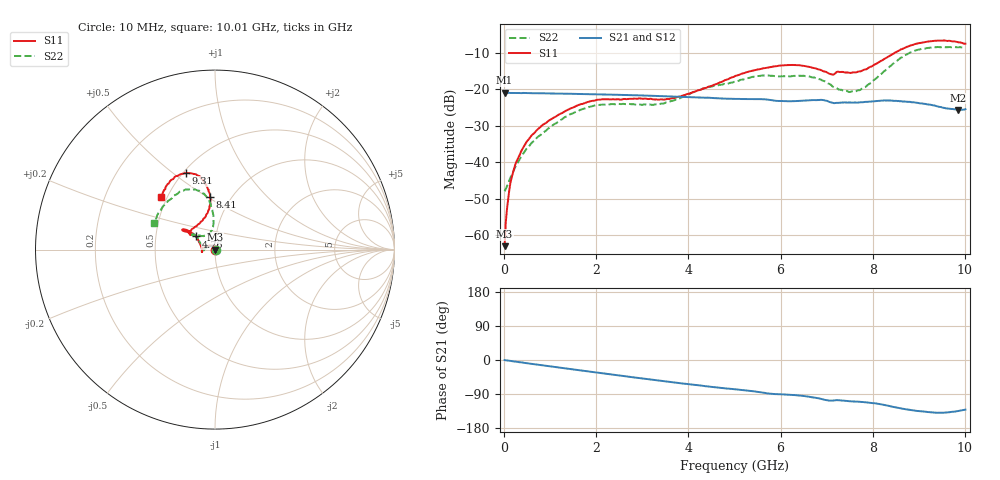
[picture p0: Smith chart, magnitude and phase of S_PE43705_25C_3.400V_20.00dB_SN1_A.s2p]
! Device ID: PE43705
! Serial: 1
! Insertion: A
! Impedance: 50 ohm
! Temp: 25C
! VDD: 3.400V
! Attenuation Step: 20.00dB
#  Hz  S  RI  R  50
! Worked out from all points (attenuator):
!   401 points, 10 MHz to 10.01 GHz, reference 50 ohm
!   highest |S21| = -21.01 dB at 10 MHz (marker M1); lowest = -25.7 dB at 9.86 GHz (marker M2)
!   lowest |S11| = -63.0 dB at 10 MHz (marker M3), VSWR 1.00, Z = 49.9 + j0.0409 ohm
!   |S11| at or under -10 dB: start of sweep to 8.485 GHz
!   |S22| runs from -48.0 to -8.5 dB; largest |S21 - S12| = 0.001
!   S11 on the Smith chart (normalised r, x): 10 MHz: 1.00, +0.00; 4.76 GHz: 0.80, +0.12; 8.41 GHz: 0.80, +0.52; 9.31 GHz: 0.52, +0.56; 10.01 GHz: 0.47, +0.33
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1e7  -0.000578 0.000409  0.089 -0.000376  0.089 -0.000338  0.00398 0.00037
8.5e7  -0.000352 0.003  0.0887 -0.00238  0.0887 -0.00237  0.00433 0.00263
1.6e8  -0.000836 0.00599  0.0886 -0.00443  0.0886 -0.00433  0.00384 0.0053
2.6e8  -0.00214 0.00974  0.0882 -0.00702  0.0881 -0.00697  0.00262 0.00864
4.35e8  -0.00587 0.0155  0.0878 -0.0116  0.0875 -0.0114  -0.000802 0.0137
8.35e8  -0.0229 0.0229  0.085 -0.0214  0.085 -0.0213  -0.016 0.0194
1.685e9  -0.0616 0.00974  0.0757 -0.04  0.0757 -0.0401  -0.0523 0.00853
2.16e9  -0.0724 -0.00493  0.0688 -0.0492  0.0687 -0.049  -0.0612 -0.00167
3.36e9  -0.0717 -0.00426  0.0468 -0.0653  0.047 -0.065  -0.0615 0.00827
4.76e9  -0.1062 0.0735  0.0202 -0.0716  0.0203 -0.0715  -0.097 0.0652
5.01e9  -0.1218 0.0884  0.0159 -0.0719  0.0162 -0.0718  -0.1045 0.0727
5.985e9  -0.1769 0.1131  -0.000391 -0.0685  -0.000115 -0.0684  -0.1197 0.0892
6.685e9  -0.1686 0.1009  -0.0104 -0.0699  -0.0101 -0.0699  -0.1201 0.0808
7.11e9  -0.1336 0.0862  -0.0195 -0.0625  -0.0191 -0.0624  -0.081 0.0768
7.585e9  -0.0938 0.1415  -0.0218 -0.0615  -0.0216 -0.0615  -0.0363 0.0849
7.885e9  -0.0524 0.1838  -0.0253 -0.062  -0.0251 -0.0622  -0.0165 0.1124
8.36e9  -0.0254 0.2836  -0.0363 -0.0596  -0.0364 -0.0597  -0.0116 0.202
8.41e9  -0.0282 0.2952  -0.0376 -0.0585  -0.0379 -0.0588  -0.0145 0.2127
8.86e9  -0.0774 0.3957  -0.0446 -0.0488  -0.0439 -0.0488  -0.0734 0.3167
9.31e9  -0.1628 0.4266  -0.0448 -0.0396  -0.0447 -0.0398  -0.1704 0.3319
9.86e9  -0.2767 0.3369  -0.0362 -0.0369  -0.0364 -0.0371  -0.3075 0.2117
1.001e10  -0.2995 0.292  -0.0349 -0.0401  -0.0347 -0.0399  -0.3408 0.15
